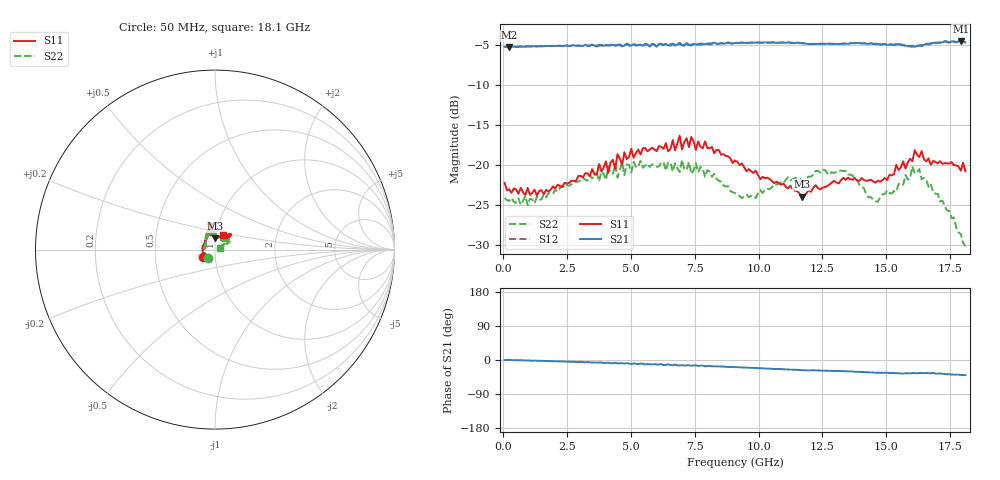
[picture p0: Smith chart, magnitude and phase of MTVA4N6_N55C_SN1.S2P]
! Network Analyzer HP8720D.06.14 Serial No. US36140669
! 28 Jun 2005  13:42:48
! Frequency  S11  S21  S12  S22
# HZ  S  DB R 50
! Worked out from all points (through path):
!   201 points, 50 MHz to 18.1 GHz, reference 50 ohm
!   highest |S21| = -4.58 dB at 17.92 GHz (marker M1); lowest = -5.3 dB at 230.5 MHz (marker M2)
!   group delay of S21, straight-line fit = 6.35 ps
!   lowest |S11| = -24.0 dB at 11.69 GHz (marker M3), VSWR 1.13, Z = 49.8 + j6.31 ohm
!   |S11| at or under -10 dB: start of sweep to end of sweep
!   |S22| runs from -30.2 to -19.4 dB; largest |S21 - S12| = 0.02
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5e7  -22.29 -148.2  -5.28 -0.4  -5.29 -0.1  -24.17 -128.9
2.305e8  -23.09 -173.4  -5.34 0.3  -5.34 0.0  -24.54 -174.3
1.3135e9  -23.88 156.7  -5.24 -1.9  -5.21 -2.0  -24.04 152.3
3.1185e9  -21.59 122.3  -5.17 -5.5  -5.17 -5.8  -21.64 129.9
6.09675e9  -17.68 99.8  -4.91 -11.9  -4.88 -11.9  -20.22 104.4
6.63825e9  -16.93 100.0  -4.88 -13.6  -4.98 -12.8  -20.85 99.2
6.7285e9  -18.22 103.1  -5.02 -11.8  -5.15 -13.0  -19.83 97.4
6.909e9  -16.38 100.8  -4.78 -14.5  -4.94 -13.7  -20.92 94.1
6.99925e9  -18.10 99.6  -5.10 -13.6  -5.11 -15.1  -19.41 95.7
7.36025e9  -16.55 93.4  -5.13 -15.3  -4.99 -14.3  -21.16 98.9
7.54075e9  -18.17 94.4  -5.00 -14.0  -4.84 -15.7  -19.80 98.5
7.90175e9  -17.10 100.7  -4.95 -16.5  -4.92 -15.5  -21.53 91.2
9.075e9  -19.49 107.6  -4.80 -18.8  -4.79 -18.9  -23.55 77.2
1.169225e10  -23.99 88.3  -4.84 -26.9  -4.83 -26.9  -22.10 52.6
1.21435e10  -22.87 83.4  -4.93 -27.0  -4.89 -27.4  -21.21 56.8
1.3407e10  -21.91 62.9  -4.88 -29.6  -4.85 -29.9  -20.82 53.6
1.458025e10  -22.25 41.9  -4.95 -33.6  -4.89 -33.9  -24.59 50.6
1.512175e10  -21.30 41.3  -5.01 -34.5  -4.91 -34.4  -23.54 46.1
1.61145e10  -18.20 44.1  -5.28 -34.5  -5.04 -35.0  -21.10 37.6
1.6295e10  -19.05 40.4  -5.14 -34.2  -5.10 -36.0  -20.56 29.0
1.79195e10  -20.75 60.2  -4.58 -39.4  -4.49 -39.1  -28.68 34.3
1.81e10  -20.82 59.8  -4.73 -39.6  -4.75 -40.5  -30.19 17.9
